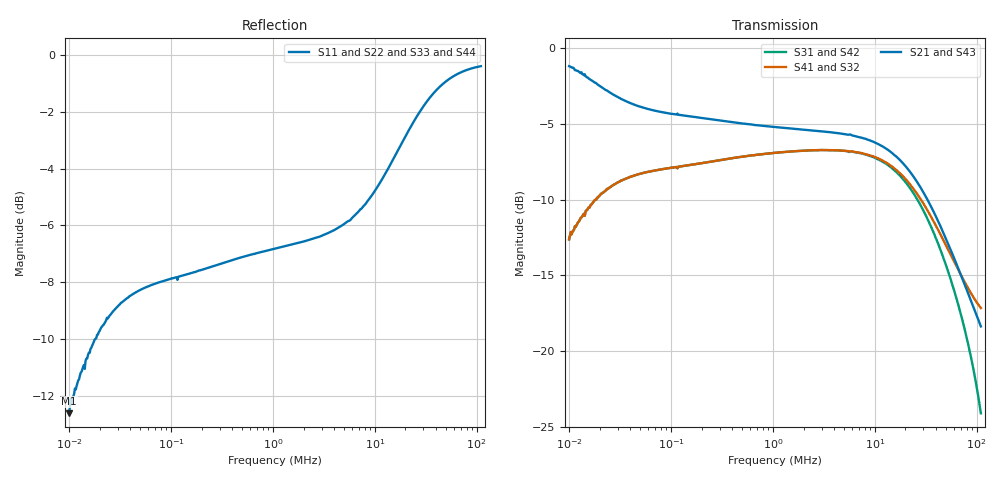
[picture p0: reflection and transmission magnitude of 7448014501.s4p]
! Touchstone file was created by TriD Version 2018.1.0 (64-bit) (07.02.2018)
! (C) EMCoS 1999-2018
! Project : TRID_WE_CMBNC_744_801_450_1_Task 1\Task 1.in
! Date  : 2018-06-17  23:47:44
# HZ S RI R  50.00
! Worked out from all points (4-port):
!   503 points, 10 kHz to 110 MHz, reference 50 ohm
!   strongest paths, dB at 10 kHz, 101.6 kHz, 1.05 MHz, 10.85 MHz, 110 MHz:
!     S21: -1.2, -4.3, -5.2, -6.3, -18.4
!     S43: -1.2, -4.3, -5.2, -6.3, -18.4
!     S41: -12.6, -7.9, -6.9, -7.3, -17.2
!     S32: -12.6, -7.9, -6.9, -7.3, -17.2
!     S31: -12.6, -7.9, -6.9, -7.3, -24.1
!     S42: -12.6, -7.9, -6.9, -7.3, -23.1
!   lowest |S11| = -12.6 dB at 10 kHz (marker M1), VSWR 1.61, Z = 62.1 + j23.9 ohm
!   |S11| at or under -10 dB: start of sweep to 18.1 kHz
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10000  0.1469 0.1818  0.8531 -0.1818  0.1467 0.1875  -0.1467 -0.1875
       0.853 -0.1818  0.147 0.1818  -0.1467 -0.1875  0.1467 0.1875
       0.1468 0.182  -0.1468 -0.182  0.147 0.1875  0.853 -0.1875
       -0.1468 -0.182  0.1468 0.182  0.853 -0.1875  0.147 0.1875
71437  0.386 0.0893  0.614 -0.0894  0.3859 0.0863  -0.3859 -0.0862
       0.614 -0.0894  0.386 0.0893  -0.3859 -0.0862  0.3859 0.0863
       0.386 0.0864  -0.386 -0.0864  0.386 0.0892  0.614 -0.0892
       -0.386 -0.0864  0.386 0.0864  0.614 -0.0892  0.386 0.0892
1492700  0.4598 0.055  0.5402 -0.0563  0.4559 -0.00413  -0.4559 0.0051
         0.5402 -0.0563  0.4598 0.0551  -0.456 0.00512  0.456 -0.00415
         0.4559 -0.00422  -0.4559 0.00519  0.4599 0.0551  0.5401 -0.0564
         -0.4559 0.00521  0.4559 -0.00424  0.5402 -0.0564  0.4598 0.0552
9885600  0.547 0.1761  0.4531 -0.1844  0.4056 -0.1582  -0.4057 0.1647
         0.4532 -0.1844  0.5467 0.1762  -0.4057 0.1647  0.4059 -0.1583
         0.4058 -0.1582  -0.4058 0.1647  0.5468 0.1762  0.4532 -0.1844
         -0.4059 0.1647  0.4061 -0.1583  0.4533 -0.1844  0.5466 0.1762
3.7544e7  0.8314 0.2037  0.1683 -0.2359  0.1327 -0.2089  -0.1324 0.2344
          0.1683 -0.2359  0.8303 0.2057  -0.1324 0.2344  0.1338 -0.2108
          0.1327 -0.2089  -0.1324 0.2344  0.8314 0.2038  0.1683 -0.2359
          -0.1324 0.2344  0.1338 -0.2108  0.1683 -0.2359  0.8303 0.2057
6.9209e7  0.9258 0.1051  0.0718 -0.1652  0.0411 -0.1276  -0.0388 0.1755
          0.0718 -0.1652  0.9247 0.1097  -0.0388 0.1754  0.0423 -0.1322
          0.0411 -0.1276  -0.0388 0.1754  0.9258 0.1052  0.0718 -0.1652
          -0.0388 0.1755  0.0423 -0.1322  0.0718 -0.1652  0.9247 0.1096
1.1e8  0.9561 0.0181  0.0362 -0.1151  0.012 -0.0612  -0.00455 0.1387
       0.0362 -0.1151  0.9556 0.0262  -0.00458 0.1385  0.0125 -0.0692
       0.012 -0.0612  -0.00458 0.1385  0.9561 0.0184  0.0362 -0.1152
       -0.00455 0.1387  0.0125 -0.0692  0.0362 -0.1152  0.9556 0.0261
